(* Logix 5000 AddOnInstructionDefinition export AMP_Tuning_Params_Servo; software revision 20.04 *)

ADD_ON_INSTRUCTION AMP_Tuning_Params_Servo   (* revision 1.0 *)
// Applied Motion - Tuning Parameters Servo AOI
// Help:
// The Tuning Parameters for Servo AOI accepts all the required parameters for SCL commands KP, KF, KD, KV, KI, KK, KE and KC, and then scales and issues these to the drive, one at a time.
VAR_IN_OUT
   MSG_Write : SINT[8]; {required}   // Message Write data tag
        [0]   // Message Reserved = 0
        [1]   // Message Type (16#01 or 16#02)
        [2]   // Type 1: Register Type 2: Opcode
        [3]   // Type 1: Opcode Type 2: Operand
        [4]   // Type 1: Parameter 1 Type 2: data MSB
        [5]   // Type 1: Parameter 2 Type 2: data LSB
        [6]   // Type 1: Parameter 3 Type 2: not used
        [7]   // Type 1: Parameter 4 Type 2: not used
   SendMsg : MESSAGE; {required}   // Message tag
   MSG_Response : SINT[8]; {required}   // Message Response data tag
        [0]   // Command Word
        [1]   // Jog Speed (0.25 rev/min)
        [2]   // Jog Acceleration (10 rev/s/s)
        [3]   // Jog Deceleration (10 rev/s/s)
        [4]   // Point-to-Point Velocity (0.25 rev/min)
        [5]   // Point-to-Point Acceleration (10 rev/s/s)
        [6]   // Point-to-Point Deceleration (10 rev/s/s)
        [7]   // Point-to-Point Distance (Motor steps)
        [9]   // (2x ASCII Letters in 16 lower word)
        [10]   // Data/Register 1
        [11]   // Data/Register 2
END_VAR
VAR_INPUT
   Configure : BOOL; {required}   // Start the Configuration
   KP : INT; {required}   // Proportional Global Gain Value
   KF : INT; {required}   // Velocity Forward Constant
   KD : INT; {required}   // Damping Gain Value
   KV : INT; {required}   // Velocity Feedback Constant
   KI : INT; {required}   // Integrator Constant
   KK : INT; {required}   // Inertia Feedforward Gain
   KE : INT; {required}   // Differential Filter Gain Value
   KC : INT; {required}   // Overall Servo Filter value
END_VAR
VAR_OUTPUT
   Sent : BOOL; {access Read Only, visible}   // All parameter settings have been sent to drive
   In_Progress : BOOL; {access Read Only, visible}   // The setting of parameters is in progress
   Done : BOOL; {access Read Only, visible}   // Parameters set without errors
   Error : BOOL; {access Read Only, visible}   // Configuration failed to complete - drive not ready or faulted
   State : DINT := 34; {access Read Only}   // Internal state of progress
END_VAR
VAR
   Loc_Start_ONS : BOOL; {access None}
   MSG_Active : BOOL;
END_VAR

ROUTINE Logic   (* ladder *)
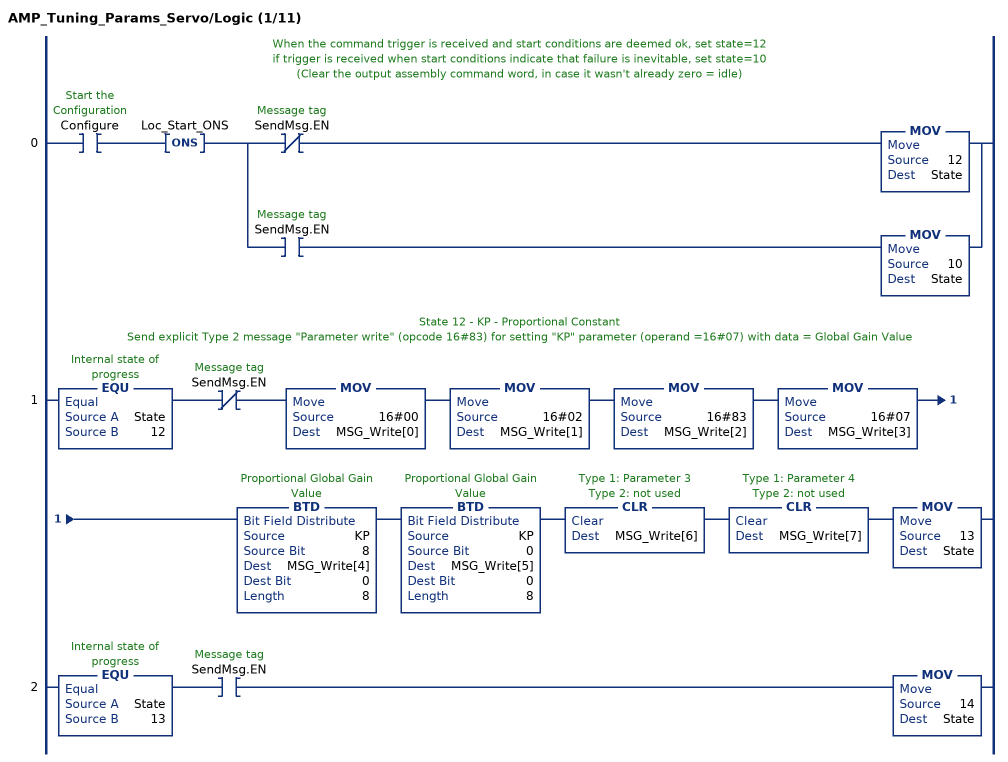
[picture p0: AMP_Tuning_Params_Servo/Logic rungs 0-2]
   // When the command trigger is received and start conditions are deemed ok, set state=12
   // if trigger is received when start conditions indicate that failure is inevitable, set state=10
   // (Clear the output assembly command word, in case it wasn't already zero = idle)
   0: XIC(Configure)ONS(Loc_Start_ONS)[XIO(SendMsg.EN) MOV(12,State) ,XIC(SendMsg.EN) MOV(10,State) ];
   // State 12 - KP - Proportional Constant
   // Send explicit Type 2 message "Parameter write" (opcode 16#83) for setting "KP" parameter (operand =16#07) with data = Global Gain Value
   1: EQU(State,12)XIO(SendMsg.EN)MOV(16#00,MSG_Write[0])MOV(16#02,MSG_Write[1])MOV(16#83,MSG_Write[2])MOV(16#07,MSG_Write[3])BTD(KP,8,MSG_Write[4],0,8)BTD(KP,0,MSG_Write[5],0,8)CLR(MSG_Write[6])CLR(MSG_Write[7])MOV(13,State);
   2: EQU(State,13)XIC(SendMsg.EN)MOV(14,State);
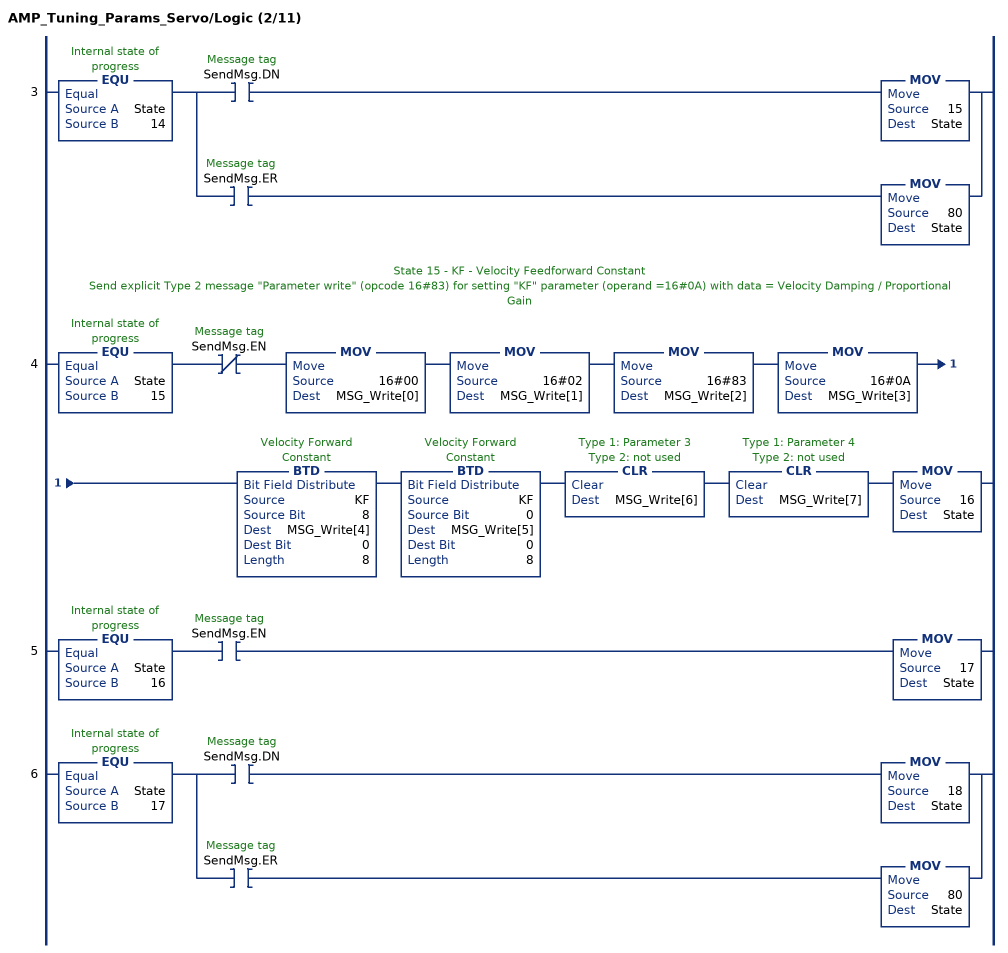
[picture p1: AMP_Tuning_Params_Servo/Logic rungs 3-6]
   3: EQU(State,14)[XIC(SendMsg.DN) MOV(15,State) ,XIC(SendMsg.ER) MOV(80,State) ];
   // State 15 - KF - Velocity Feedforward Constant
   // Send explicit Type 2 message "Parameter write" (opcode 16#83) for setting "KF" parameter (operand =16#0A) with data = Velocity Damping / Proportional Gain
   4: EQU(State,15)XIO(SendMsg.EN)MOV(16#00,MSG_Write[0])MOV(16#02,MSG_Write[1])MOV(16#83,MSG_Write[2])MOV(16#0A,MSG_Write[3])BTD(KF,8,MSG_Write[4],0,8)BTD(KF,0,MSG_Write[5],0,8)CLR(MSG_Write[6])CLR(MSG_Write[7])MOV(16,State);
   5: EQU(State,16)XIC(SendMsg.EN)MOV(17,State);
   6: EQU(State,17)[XIC(SendMsg.DN) MOV(18,State) ,XIC(SendMsg.ER) MOV(80,State) ];
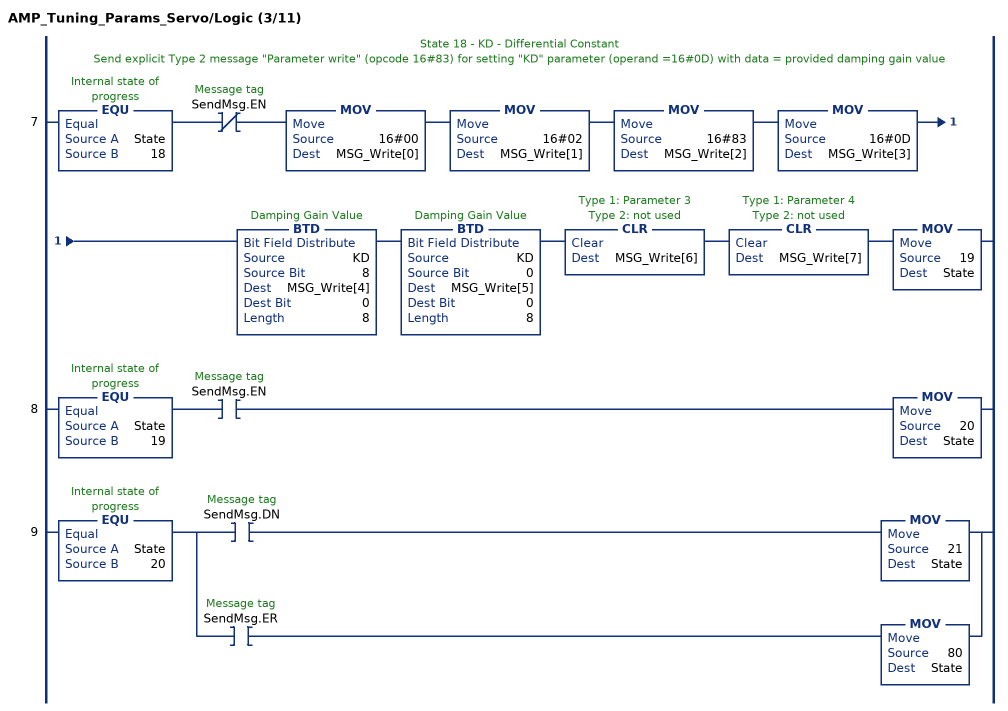
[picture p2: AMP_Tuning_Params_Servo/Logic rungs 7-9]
   // State 18 - KD - Differential Constant
   // Send explicit Type 2 message "Parameter write" (opcode 16#83) for setting "KD" parameter (operand =16#0D) with data = provided damping gain value
   7: EQU(State,18)XIO(SendMsg.EN)MOV(16#00,MSG_Write[0])MOV(16#02,MSG_Write[1])MOV(16#83,MSG_Write[2])MOV(16#0D,MSG_Write[3])BTD(KD,8,MSG_Write[4],0,8)BTD(KD,0,MSG_Write[5],0,8)CLR(MSG_Write[6])CLR(MSG_Write[7])MOV(19,State);
   8: EQU(State,19)XIC(SendMsg.EN)MOV(20,State);
   9: EQU(State,20)[XIC(SendMsg.DN) MOV(21,State) ,XIC(SendMsg.ER) MOV(80,State) ];
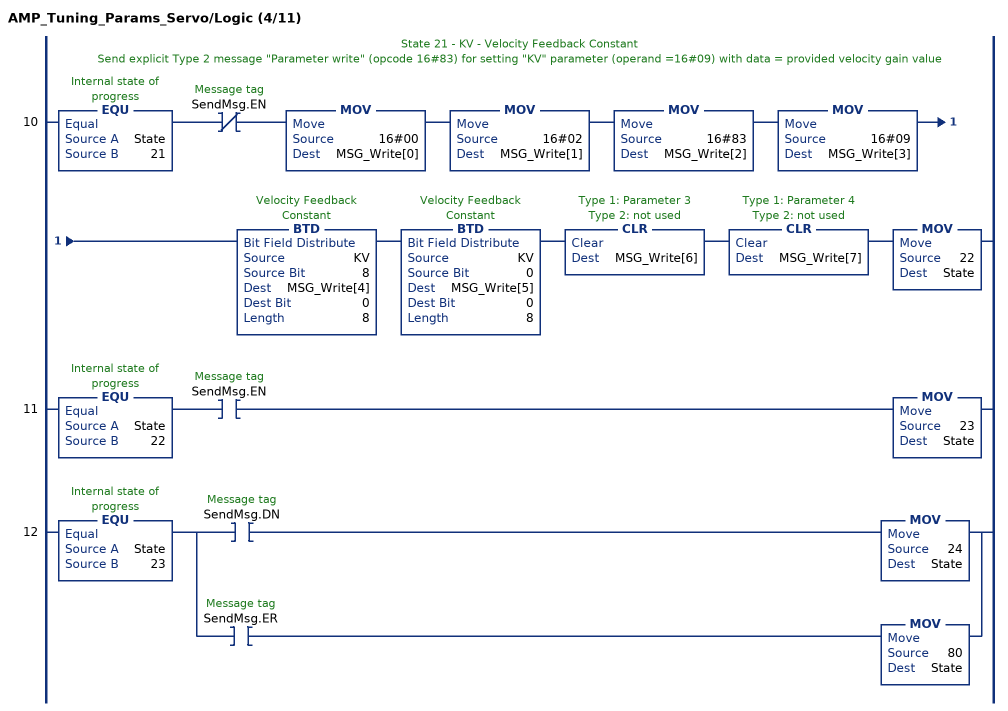
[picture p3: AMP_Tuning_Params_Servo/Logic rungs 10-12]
   // State 21 - KV - Velocity Feedback Constant
   // Send explicit Type 2 message "Parameter write" (opcode 16#83) for setting "KV" parameter (operand =16#09) with data = provided velocity gain value
   10: EQU(State,21)XIO(SendMsg.EN)MOV(16#00,MSG_Write[0])MOV(16#02,MSG_Write[1])MOV(16#83,MSG_Write[2])MOV(16#09,MSG_Write[3])BTD(KV,8,MSG_Write[4],0,8)BTD(KV,0,MSG_Write[5],0,8)CLR(MSG_Write[6])CLR(MSG_Write[7])MOV(22,State);
   11: EQU(State,22)XIC(SendMsg.EN)MOV(23,State);
   12: EQU(State,23)[XIC(SendMsg.DN) MOV(24,State) ,XIC(SendMsg.ER) MOV(80,State) ];
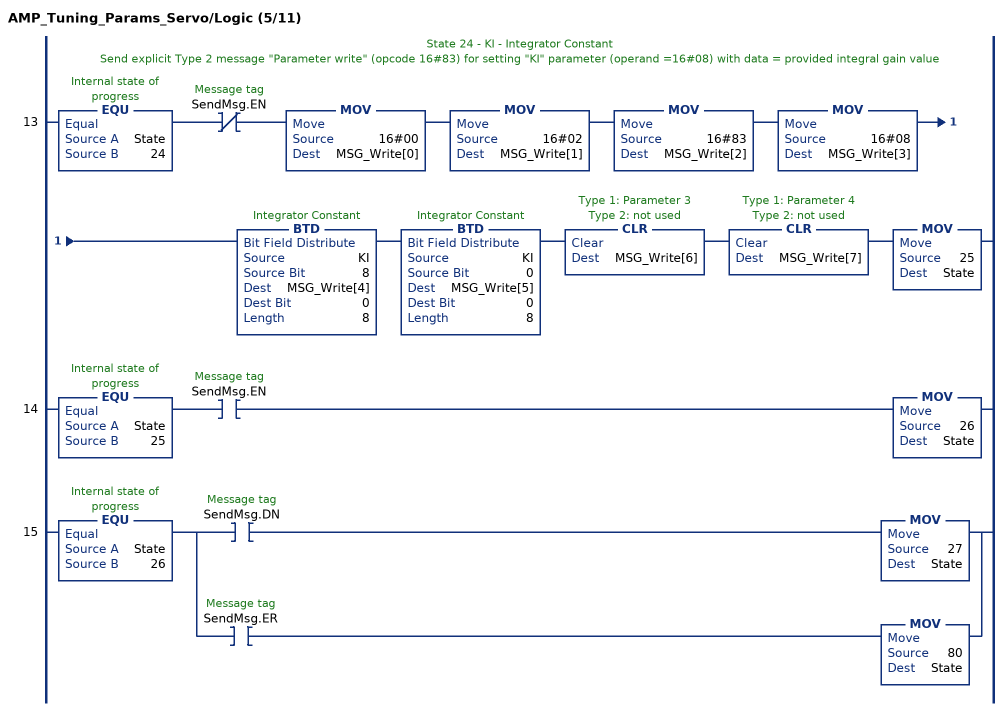
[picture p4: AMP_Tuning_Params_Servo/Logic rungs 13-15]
   // State 24 - KI - Integrator Constant
   // Send explicit Type 2 message "Parameter write" (opcode 16#83) for setting "KI" parameter (operand =16#08) with data = provided integral gain value
   13: EQU(State,24)XIO(SendMsg.EN)MOV(16#00,MSG_Write[0])MOV(16#02,MSG_Write[1])MOV(16#83,MSG_Write[2])MOV(16#08,MSG_Write[3])BTD(KI,8,MSG_Write[4],0,8)BTD(KI,0,MSG_Write[5],0,8)CLR(MSG_Write[6])CLR(MSG_Write[7])MOV(25,State);
   14: EQU(State,25)XIC(SendMsg.EN)MOV(26,State);
   15: EQU(State,26)[XIC(SendMsg.DN) MOV(27,State) ,XIC(SendMsg.ER) MOV(80,State) ];
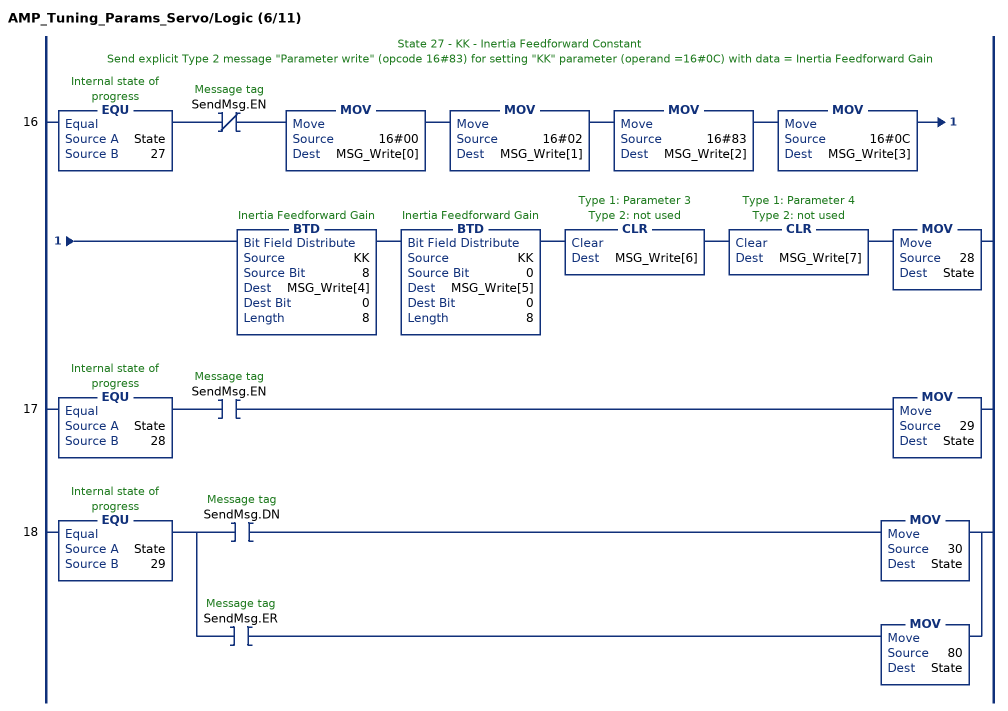
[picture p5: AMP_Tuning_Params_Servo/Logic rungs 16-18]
   // State 27 - KK - Inertia Feedforward Constant
   // Send explicit Type 2 message "Parameter write" (opcode 16#83) for setting "KK" parameter (operand =16#0C) with data = Inertia Feedforward Gain
   16: EQU(State,27)XIO(SendMsg.EN)MOV(16#00,MSG_Write[0])MOV(16#02,MSG_Write[1])MOV(16#83,MSG_Write[2])MOV(16#0C,MSG_Write[3])BTD(KK,8,MSG_Write[4],0,8)BTD(KK,0,MSG_Write[5],0,8)CLR(MSG_Write[6])CLR(MSG_Write[7])MOV(28,State);
   17: EQU(State,28)XIC(SendMsg.EN)MOV(29,State);
   18: EQU(State,29)[XIC(SendMsg.DN) MOV(30,State) ,XIC(SendMsg.ER) MOV(80,State) ];
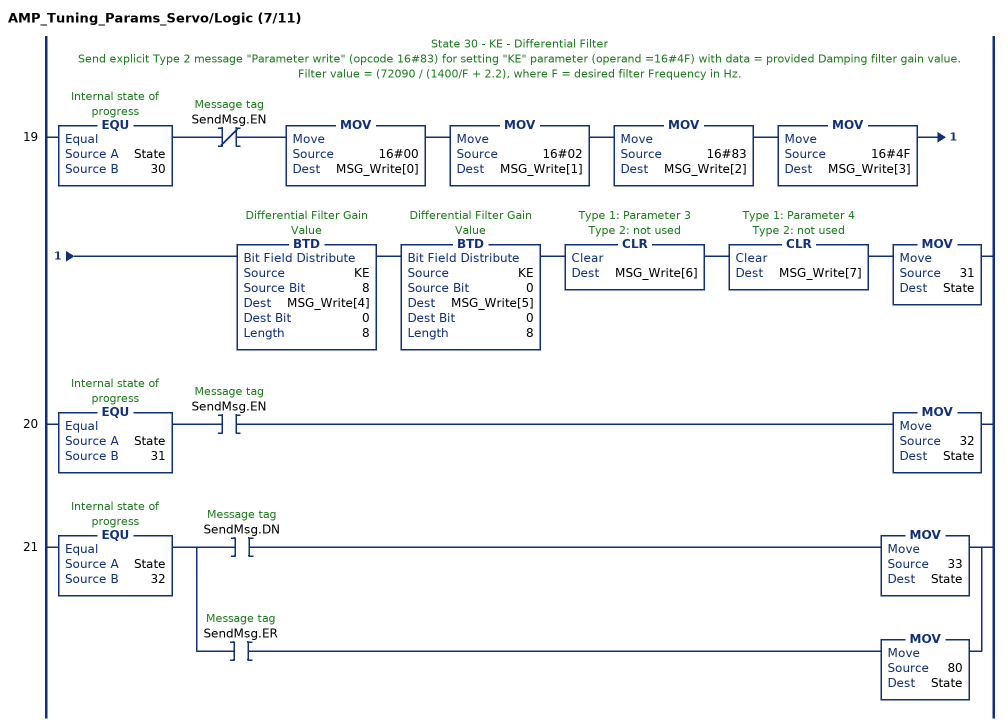
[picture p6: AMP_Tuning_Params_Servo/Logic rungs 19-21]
   // State 30 - KE - Differential Filter
   // Send explicit Type 2 message "Parameter write" (opcode 16#83) for setting "KE" parameter (operand =16#4F) with data = provided Damping filter gain value. Filter value = (72090 / (1400/F + 2.2), where F = desired filter Frequency in Hz.
   19: EQU(State,30)XIO(SendMsg.EN)MOV(16#00,MSG_Write[0])MOV(16#02,MSG_Write[1])MOV(16#83,MSG_Write[2])MOV(16#4F,MSG_Write[3])BTD(KE,8,MSG_Write[4],0,8)BTD(KE,0,MSG_Write[5],0,8)CLR(MSG_Write[6])CLR(MSG_Write[7])MOV(31,State);
   20: EQU(State,31)XIC(SendMsg.EN)MOV(32,State);
   21: EQU(State,32)[XIC(SendMsg.DN) MOV(33,State) ,XIC(SendMsg.ER) MOV(80,State) ];
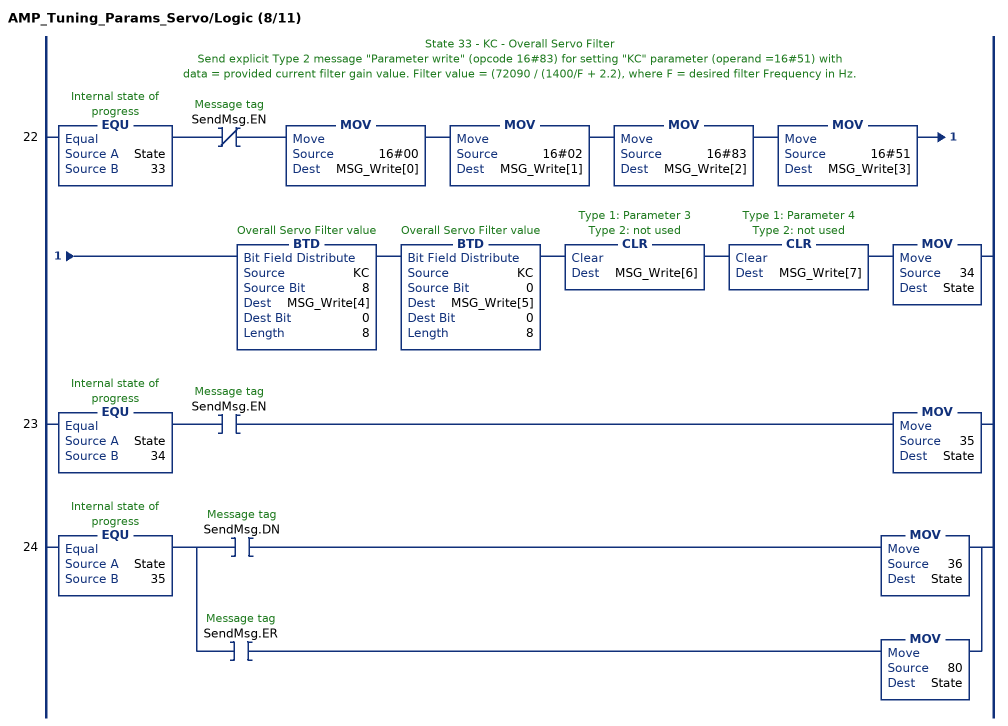
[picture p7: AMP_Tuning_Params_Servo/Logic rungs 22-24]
   // State 33 - KC - Overall Servo Filter
   // Send explicit Type 2 message "Parameter write" (opcode 16#83) for setting "KC" parameter (operand =16#51) with
   // data = provided current filter gain value. Filter value = (72090 / (1400/F + 2.2), where F = desired filter Frequency in Hz.
   22: EQU(State,33)XIO(SendMsg.EN)MOV(16#00,MSG_Write[0])MOV(16#02,MSG_Write[1])MOV(16#83,MSG_Write[2])MOV(16#51,MSG_Write[3])BTD(KC,8,MSG_Write[4],0,8)BTD(KC,0,MSG_Write[5],0,8)CLR(MSG_Write[6])CLR(MSG_Write[7])MOV(34,State);
   23: EQU(State,34)XIC(SendMsg.EN)MOV(35,State);
   24: EQU(State,35)[XIC(SendMsg.DN) MOV(36,State) ,XIC(SendMsg.ER) MOV(80,State) ];
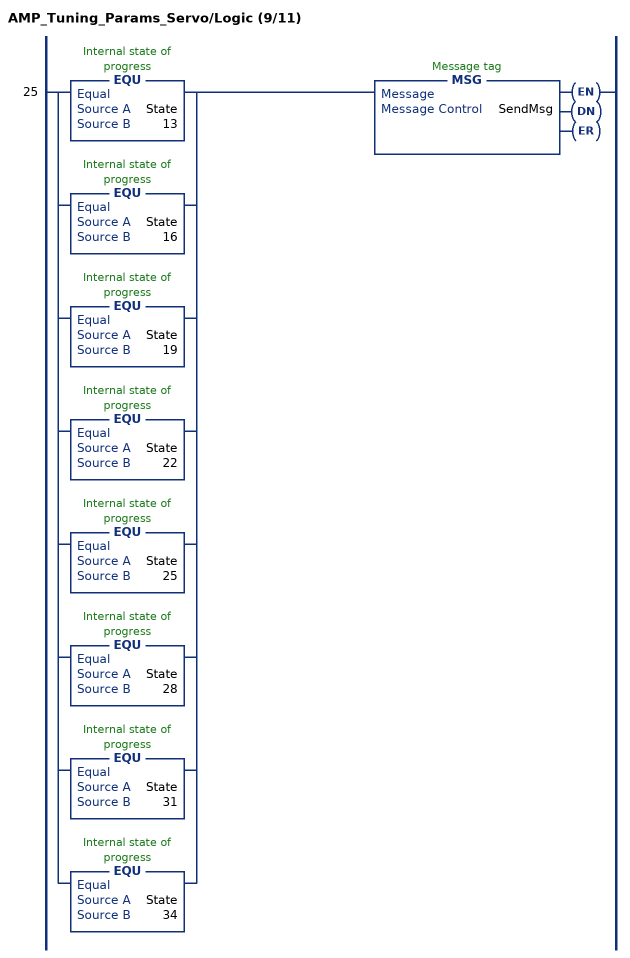
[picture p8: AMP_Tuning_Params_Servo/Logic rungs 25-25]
   25: [EQU(State,13) ,EQU(State,16) ,EQU(State,19) ,EQU(State,22) ,EQU(State,25) ,EQU(State,28) ,EQU(State,31) ,EQU(State,34) ]MSG(SendMsg);
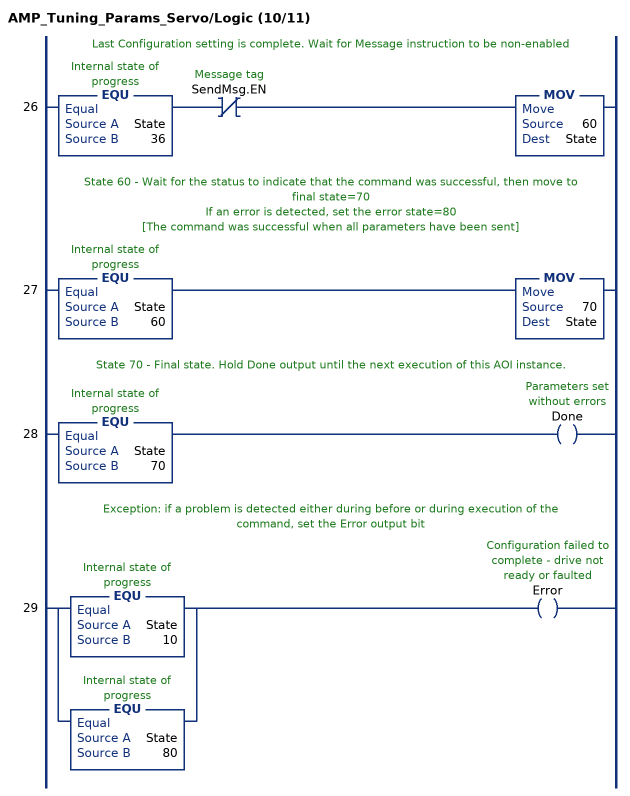
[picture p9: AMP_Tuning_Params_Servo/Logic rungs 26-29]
   // Last Configuration setting is complete. Wait for Message instruction to be non-enabled
   26: EQU(State,36)XIO(SendMsg.EN)MOV(60,State);
   // State 60 - Wait for the status to indicate that the command was successful, then move to final state=70
   // If an error is detected, set the error state=80
   // [The command was successful when all parameters have been sent]
   27: EQU(State,60)MOV(70,State);
   // State 70 - Final state. Hold Done output until the next execution of this AOI instance.
   28: EQU(State,70)OTE(Done);
   // Exception: if a problem is detected either during before or during execution of the command, set the Error output bit
   29: [EQU(State,10) ,EQU(State,80) ]OTE(Error);
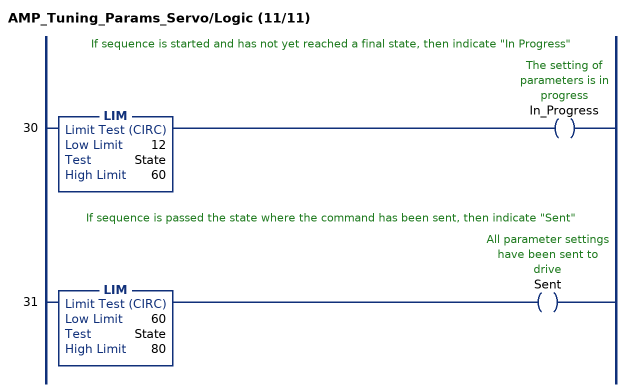
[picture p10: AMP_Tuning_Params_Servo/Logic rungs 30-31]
   // If sequence is started and has not yet reached a final state, then indicate "In Progress"
   30: LIM(12,State,60)OTE(In_Progress);
   // If sequence is passed the state where the command has been sent, then indicate "Sent"
   31: LIM(60,State,80)OTE(Sent);
END_ROUTINE
END_ADD_ON_INSTRUCTION
